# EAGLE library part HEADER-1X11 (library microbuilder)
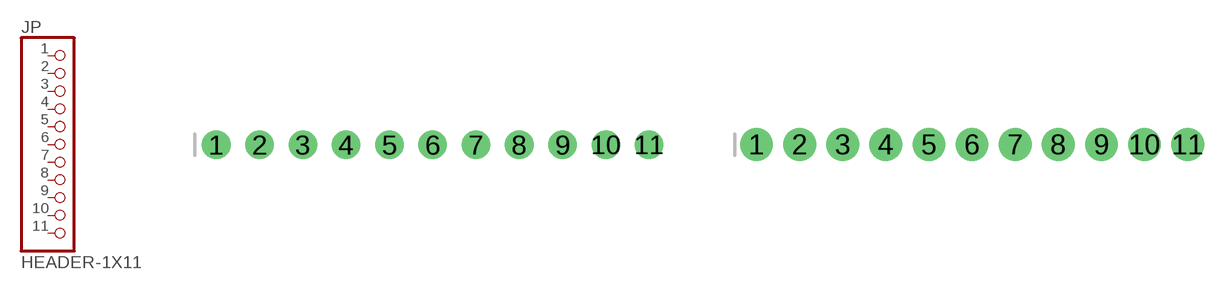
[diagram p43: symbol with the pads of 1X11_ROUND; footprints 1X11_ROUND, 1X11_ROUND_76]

Designator prefix JP

## HEADER-1X11  [1X11_ROUND]
1  1  pas
2  2  pas
3  3  pas
4  4  pas
5  5  pas
6  6  pas
7  7  pas
8  8  pas
9  9  pas
10  10  pas
11  11  pas

## HEADER-1X1176MIL  [1X11_ROUND_76]
Pads as for 1X11_ROUND

## Footprint 1X11_ROUND (pad centres in mm)
drill 1 pad 1.676: 1 -12.7,0; 2 -10.16,0; 3 -7.62,0; 4 -5.08,0; 5 -2.54,0; 6 0,0; 7 2.54,0; 8 5.08,0; 9 7.62,0; 10 10.16,0; 11 12.7,0

## Footprint 1X11_ROUND_76 (pad centres in mm)
drill 1 pad 1.93: 1 -12.7,0; 2 -10.16,0; 3 -7.62,0; 4 -5.08,0; 5 -2.54,0; 6 0,0; 7 2.54,0; 8 5.08,0; 9 7.62,0; 10 10.16,0; 11 12.7,0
